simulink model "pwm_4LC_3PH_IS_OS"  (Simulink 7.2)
settings: Solver=ode3  SolverMode=SingleTasking  StartTime=0.0  StopTime=0.1  FixedStep=10e-6  MaxStep=1e-4  RelTol=1e-3

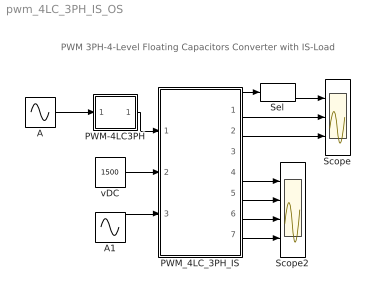
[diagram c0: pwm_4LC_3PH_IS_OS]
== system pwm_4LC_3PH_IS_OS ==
  note: PWM 3PH-4-Level Floating Capacitors Converter with IS-Load
  A : Sin  Amplitude=.9  Frequency=2*pi*50  Phase="[0  -2*pi/3  -4*pi/3]"  SampleTime=0
  A1 : Sin  Amplitude=500  Frequency=2*pi*50  Phase="[0  -2*pi/3 ]"  SampleTime=0
  PWM-4LC3PH : Subsystem  mask(PWM-4LC3PH){FT=900, PHT1=0, PHT2=-120, PHT3=-240, DT=1e-6}
      mask prompts: FT "Frequency of Trian Sig."; PHT1 "Phase Angle of 1st Trian. Sig."; PHT2 "Phase Angle of 2nd Trian. Sig."; PHT3 "Phase Angle of 3rd Trian. Sig."; DT "Dead Time"
  PWM_4LC_3PH_IS : Subsystem  mask(pwm_4LC_3PH_IS_OS){C1=10e-3, VC10=2*1500/3, C2=10e-3, VC20=1500/3}
      mask prompts: C1 "Cap C1"; VC10 "Initial Cap Voltage VC10"; C2 "Cap C2"; VC20 "Initial Cap Voltage VC20"
      mask help: Open Source 4-Level FC PWM 3PH Converter with IS load Input Vector u: u[0]= L4LC1_TD1.gate u[1]= L4LC1_TD2.gate u[2]= L4LC1_TD3.gate u[3]= L4LC1_TD4.gate u[4]= L4LC1_TD5.gate u[5]= L4LC1_TD6.gate u[6]= L4LC2_TD1.gate u[7]= L4LC2_TD2.gate u[8]= L4LC2_TD3.gate u[9]= L4LC2_TD4.gate u[10]= L4LC2_TD5.gate u[11]= L4LC2_TD6.gate u[12]= L4LC3_TD1.gate u[13]= L4LC3_TD2.gate u[14]= L4LC3_TD3.gate u[15]= L4LC3_TD4.gate u[15]= L4LC3_TD5.gate u[17]= L4LC3_TD6.gate u[18]= VDC u[19]= IA, Phase A Load Current as AC Current source u[20]= IB, Phase B Load Current as AC Current source Output Vector y: y[0]= Va.v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
  Scope : Scope  NumInputPorts=3
  Scope2 : Scope  NumInputPorts=4
  Sel : Selector  InputPortWidth=3  IndexOptions=Index vector (dialog)  Indices=[1 ]  OutputSizes=1
  vDC : Constant  Value=1500  OutDataType=sfix(16)  OutScaling=2^0
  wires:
  A/1 -> PWM-4LC3PH/1(In1)
  PWM-4LC3PH/1(Out1) -> PWM_4LC_3PH_IS/1(Sw)
  PWM_4LC_3PH_IS/1(vABC) -> Sel/1
  PWM_4LC_3PH_IS/2(iABC) -> Scope/2
  PWM_4LC_3PH_IS/3(vAB) -> Scope/3
  vDC/1 -> PWM_4LC_3PH_IS/2(vDC)
  A1/1 -> PWM_4LC_3PH_IS/3(i_AB)
  PWM_4LC_3PH_IS/4(iT1,iD1,vT1) -> Scope2/1
  PWM_4LC_3PH_IS/5(iT2,ID2,vT2) -> Scope2/2
  PWM_4LC_3PH_IS/6(iT3,iD3,vT3) -> Scope2/3
  PWM_4LC_3PH_IS/7(iDC1,IDC2) -> Scope2/4
  Sel/1 -> Scope/1

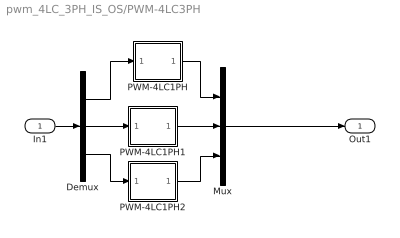
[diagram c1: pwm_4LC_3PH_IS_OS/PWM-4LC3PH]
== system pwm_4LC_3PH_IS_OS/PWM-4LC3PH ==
  In1 : Inport  OutDataType=sfix(16)  OutScaling=2^0
  Demux : Demux  Outputs=3
  Mux : Mux  Inputs=3
  PWM-4LC1PH : Subsystem  mask(PWM-4LC1PH){FT=FT, PHT1=PHT1, PHT2=PHT2, PHT3=PHT3, DT=DT}
      mask prompts: FT "Frequency of Trian Sig."; PHT1 "Phase Angle of 1st Trian. Sig."; PHT2 "Phase Angle of 2nd Trian. Sig."; PHT3 "Phase Angle of 3rd Trian. Sig."; DT "Dead Time"
      mask help: Pulse Width Modulation for 1 Phase 4 Level Floating Capacitor Converter
  PWM-4LC1PH1 : Subsystem  mask(PWM-4LC1PH){FT=FT, PHT1=PHT1, PHT2=PHT2, PHT3=PHT3, DT=DT}
      mask prompts: FT "Frequency of Trian Sig."; PHT1 "Phase Angle of 1st Trian. Sig."; PHT2 "Phase Angle of 2nd Trian. Sig."; PHT3 "Phase Angle of 3rd Trian. Sig."; DT "Dead Time"
      mask help: Pulse Width Modulation for 1 Phase 4 Level Floating Capacitor Converter
  PWM-4LC1PH2 : Subsystem  mask(PWM-4LC1PH){FT=FT, PHT1=PHT1, PHT2=PHT2, PHT3=PHT3, DT=DT}
      mask prompts: FT "Frequency of Trian Sig."; PHT1 "Phase Angle of 1st Trian. Sig."; PHT2 "Phase Angle of 2nd Trian. Sig."; PHT3 "Phase Angle of 3rd Trian. Sig."; DT "Dead Time"
      mask help: Pulse Width Modulation for 1 Phase 4 Level Floating Capacitor Converter
  Out1 : Outport
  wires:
  PWM-4LC1PH/1(Out1) -> Mux/1
  PWM-4LC1PH1/1(Out1) -> Mux/2
  PWM-4LC1PH2/1(Out1) -> Mux/3
  Demux/1 -> PWM-4LC1PH/1(In1)
  Demux/2 -> PWM-4LC1PH1/1(In1)
  Demux/3 -> PWM-4LC1PH2/1(In1)
  Mux/1 -> Out1/1
  In1/1 -> Demux/1

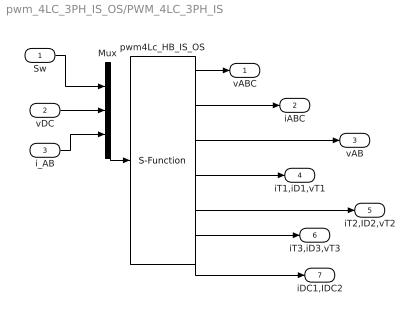
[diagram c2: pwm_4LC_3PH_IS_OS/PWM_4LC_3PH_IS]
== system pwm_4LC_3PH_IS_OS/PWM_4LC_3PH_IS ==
  Sw : Inport  OutDataType=sfix(16)  OutScaling=2^0
  vDC : Inport  Port=2  OutDataType=sfix(16)  OutScaling=2^0
  i_AB : Inport  Port=3  OutDataType=sfix(16)  OutScaling=2^0
  Mux : Mux  Inputs="[18  1  2]"
  pwm4Lc_HB_IS_OS : S-Function  FunctionName=s_pwm_4LC_3PH_IS_OS  Parameters="[C1  VC10  C2  VC20]"  EnableBusSupport=off
  vABC : Outport  OutDataType=sfix(16)  OutScaling=2^0
  iABC : Outport  Port=2  OutDataType=sfix(16)  OutScaling=2^0
  vAB : Outport  Port=3  OutDataType=sfix(16)  OutScaling=2^0
  iT1,iD1,vT1 : Outport  Port=4  OutDataType=sfix(16)  OutScaling=2^0
  iT2,ID2,vT2 : Outport  Port=5  OutDataType=sfix(16)  OutScaling=2^0
  iT3,iD3,vT3 : Outport  Port=6  OutDataType=sfix(16)  OutScaling=2^0
  iDC1,IDC2 : Outport  Port=7  OutDataType=sfix(16)  OutScaling=2^0
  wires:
  pwm4Lc_HB_IS_OS/7 -> iDC1,IDC2/1
  pwm4Lc_HB_IS_OS/2 -> iABC/1
  pwm4Lc_HB_IS_OS/1 -> vABC/1
  i_AB/1 -> Mux/3
  Mux/1 -> pwm4Lc_HB_IS_OS/1
  vDC/1 -> Mux/2
  Sw/1 -> Mux/1
  pwm4Lc_HB_IS_OS/3 -> vAB/1
  pwm4Lc_HB_IS_OS/4 -> iT1,iD1,vT1/1
  pwm4Lc_HB_IS_OS/5 -> iT2,ID2,vT2/1
  pwm4Lc_HB_IS_OS/6 -> iT3,iD3,vT3/1

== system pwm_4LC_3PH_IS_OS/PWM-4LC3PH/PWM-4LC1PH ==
  In1 : Inport  OutDataType=sfix(16)  OutScaling=2^0
  Mux : Mux  Inputs=6
  PWM-2L-1PH : Subsystem  mask(PWM-2L-1PH){FT=FT, PHT=PHT1, DT=DT}
      mask prompts: FT "Triangular Frequency"; PHT "Trian. Phase Angle (Degree)"; DT "Dead Time"
      mask help: Pulse Width Modulation for 1 Phase Converter
  PWM-2L-1PH1 : Subsystem  mask(PWM-2L-1PH){FT=FT, PHT=PHT2, DT=DT}
      mask prompts: FT "Triangular Frequency"; PHT "Trian. Phase Angle (Degree)"; DT "Dead Time"
      mask help: Pulse Width Modulation for 1 Phase Converter
  PWM-2L-1PH2 : Subsystem  mask(PWM-2L-1PH){FT=FT, PHT=PHT3, DT=DT}
      mask prompts: FT "Triangular Frequency"; PHT "Trian. Phase Angle (Degree)"; DT "Dead Time"
      mask help: Pulse Width Modulation for 1 Phase Converter
  Out1 : Outport
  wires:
  PWM-2L-1PH/1(Out1) -> Mux/1
  PWM-2L-1PH1/1(Out1) -> Mux/2
  PWM-2L-1PH1/2(Out2) -> Mux/5
  PWM-2L-1PH2/1(Out1) -> Mux/3
  PWM-2L-1PH2/2(Out2) -> Mux/4
  Mux/1 -> Out1/1
  In1/1 -> PWM-2L-1PH2/1(In1), PWM-2L-1PH1/1(In1), PWM-2L-1PH/1(In1)
  PWM-2L-1PH/2(Out2) -> Mux/6

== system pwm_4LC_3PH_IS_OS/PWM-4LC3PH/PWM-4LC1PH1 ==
  In1 : Inport  OutDataType=sfix(16)  OutScaling=2^0
  Mux : Mux  Inputs=6
  PWM-2L-1PH : Subsystem  mask(PWM-2L-1PH){FT=FT, PHT=PHT1, DT=DT}
      mask prompts: FT "Triangular Frequency"; PHT "Trian. Phase Angle (Degree)"; DT "Dead Time"
      mask help: Pulse Width Modulation for 1 Phase Converter
  PWM-2L-1PH1 : Subsystem  mask(PWM-2L-1PH){FT=FT, PHT=PHT2, DT=DT}
      mask prompts: FT "Triangular Frequency"; PHT "Trian. Phase Angle (Degree)"; DT "Dead Time"
      mask help: Pulse Width Modulation for 1 Phase Converter
  PWM-2L-1PH2 : Subsystem  mask(PWM-2L-1PH){FT=FT, PHT=PHT3, DT=DT}
      mask prompts: FT "Triangular Frequency"; PHT "Trian. Phase Angle (Degree)"; DT "Dead Time"
      mask help: Pulse Width Modulation for 1 Phase Converter
  Out1 : Outport
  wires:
  PWM-2L-1PH/2(Out2) -> Mux/6
  In1/1 -> PWM-2L-1PH/1(In1), PWM-2L-1PH1/1(In1), PWM-2L-1PH2/1(In1)
  Mux/1 -> Out1/1
  PWM-2L-1PH2/2(Out2) -> Mux/4
  PWM-2L-1PH2/1(Out1) -> Mux/3
  PWM-2L-1PH1/2(Out2) -> Mux/5
  PWM-2L-1PH1/1(Out1) -> Mux/2
  PWM-2L-1PH/1(Out1) -> Mux/1

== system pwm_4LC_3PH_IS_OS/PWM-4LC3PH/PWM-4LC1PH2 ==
  In1 : Inport  OutDataType=sfix(16)  OutScaling=2^0
  Mux : Mux  Inputs=6
  PWM-2L-1PH : Subsystem  mask(PWM-2L-1PH){FT=FT, PHT=PHT1, DT=DT}
      mask prompts: FT "Triangular Frequency"; PHT "Trian. Phase Angle (Degree)"; DT "Dead Time"
      mask help: Pulse Width Modulation for 1 Phase Converter
  PWM-2L-1PH1 : Subsystem  mask(PWM-2L-1PH){FT=FT, PHT=PHT2, DT=DT}
      mask prompts: FT "Triangular Frequency"; PHT "Trian. Phase Angle (Degree)"; DT "Dead Time"
      mask help: Pulse Width Modulation for 1 Phase Converter
  PWM-2L-1PH2 : Subsystem  mask(PWM-2L-1PH){FT=FT, PHT=PHT3, DT=DT}
      mask prompts: FT "Triangular Frequency"; PHT "Trian. Phase Angle (Degree)"; DT "Dead Time"
      mask help: Pulse Width Modulation for 1 Phase Converter
  Out1 : Outport
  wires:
  PWM-2L-1PH/1(Out1) -> Mux/1
  PWM-2L-1PH1/1(Out1) -> Mux/2
  PWM-2L-1PH1/2(Out2) -> Mux/5
  PWM-2L-1PH2/1(Out1) -> Mux/3
  PWM-2L-1PH2/2(Out2) -> Mux/4
  Mux/1 -> Out1/1
  In1/1 -> PWM-2L-1PH2/1(In1), PWM-2L-1PH1/1(In1), PWM-2L-1PH/1(In1)
  PWM-2L-1PH/2(Out2) -> Mux/6

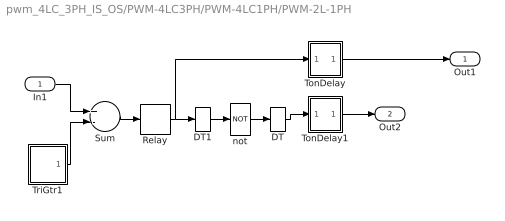
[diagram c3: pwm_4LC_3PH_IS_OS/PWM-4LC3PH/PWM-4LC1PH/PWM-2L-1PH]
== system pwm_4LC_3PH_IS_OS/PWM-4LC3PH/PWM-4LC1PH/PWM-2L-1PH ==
  In1 : Inport  OutDataType=sfix(16)  OutScaling=2^0
  DT : DataTypeConversion
  DT1 : DataTypeConversion
  Relay : Relay  OutDataType=sfix(16)  OutScaling=2^0
  Sum : Sum  Inputs=+-  OutDataType=sfix(16)  OutScaling=2^0
  TonDelay : Subsystem  mask(TonDelay){DT=DT}
      mask prompts: DT "Dead Time"
      mask help: Turn on dead time to protect against short circuit of the converter leg
  TonDelay1 : Subsystem  mask(TonDelay){DT=DT}
      mask prompts: DT "Dead Time"
      mask help: Turn on dead time to protect against short circuit of the converter leg
  TriGtr1 : Subsystem  mask(TriGtr){T=1/FT, Td=PHT/FT/360}
      mask prompts: T "Period Time"; Td "Time Delay"
      mask help: Triangular Wave Generator with variable time delay
  not : Logic  Operator=NOT  Inputs=1
  Out1 : Outport  InitialOutput=0
  Out2 : Outport  Port=2  InitialOutput=0
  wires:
  DT1/1 -> not/1
  DT/1 -> TonDelay1/1(s1)
  In1/1 -> Sum/1
  TriGtr1/1(O) -> Sum/2
  Sum/1 -> Relay/1
  not/1 -> DT/1
  TonDelay1/1(s1d) -> Out2/1
  Relay/1 -> DT1/1, TonDelay/1(s1)
  TonDelay/1(s1d) -> Out1/1

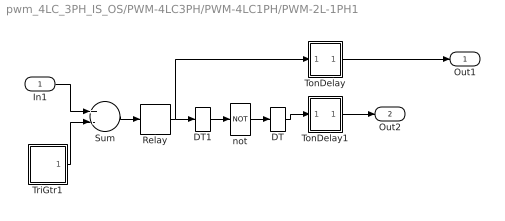
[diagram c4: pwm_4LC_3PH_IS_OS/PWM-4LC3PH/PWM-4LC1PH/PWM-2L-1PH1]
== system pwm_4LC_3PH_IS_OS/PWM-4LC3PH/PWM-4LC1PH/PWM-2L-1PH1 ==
  In1 : Inport  OutDataType=sfix(16)  OutScaling=2^0
  DT : DataTypeConversion
  DT1 : DataTypeConversion
  Relay : Relay  OutDataType=sfix(16)  OutScaling=2^0
  Sum : Sum  Inputs=+-  OutDataType=sfix(16)  OutScaling=2^0
  TonDelay : Subsystem  mask(TonDelay){DT=DT}
      mask prompts: DT "Dead Time"
      mask help: Turn on dead time to protect against short circuit of the converter leg
  TonDelay1 : Subsystem  mask(TonDelay){DT=DT}
      mask prompts: DT "Dead Time"
      mask help: Turn on dead time to protect against short circuit of the converter leg
  TriGtr1 : Subsystem  mask(TriGtr){T=1/FT, Td=PHT/FT/360}
      mask prompts: T "Period Time"; Td "Time Delay"
      mask help: Triangular Wave Generator with variable time delay
  not : Logic  Operator=NOT  Inputs=1
  Out1 : Outport  InitialOutput=0
  Out2 : Outport  Port=2  InitialOutput=0
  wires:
  TonDelay/1(s1d) -> Out1/1
  Relay/1 -> TonDelay/1(s1), DT1/1
  TonDelay1/1(s1d) -> Out2/1
  not/1 -> DT/1
  Sum/1 -> Relay/1
  TriGtr1/1(O) -> Sum/2
  In1/1 -> Sum/1
  DT/1 -> TonDelay1/1(s1)
  DT1/1 -> not/1

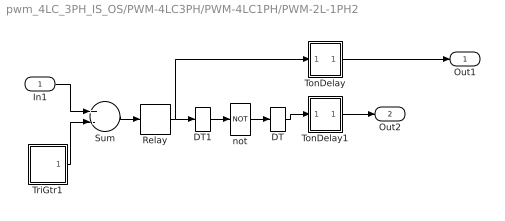
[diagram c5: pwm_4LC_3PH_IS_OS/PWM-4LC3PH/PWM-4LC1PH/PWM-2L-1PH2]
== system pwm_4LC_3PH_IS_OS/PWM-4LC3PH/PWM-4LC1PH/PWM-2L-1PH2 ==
  In1 : Inport  OutDataType=sfix(16)  OutScaling=2^0
  DT : DataTypeConversion
  DT1 : DataTypeConversion
  Relay : Relay  OutDataType=sfix(16)  OutScaling=2^0
  Sum : Sum  Inputs=+-  OutDataType=sfix(16)  OutScaling=2^0
  TonDelay : Subsystem  mask(TonDelay){DT=DT}
      mask prompts: DT "Dead Time"
      mask help: Turn on dead time to protect against short circuit of the converter leg
  TonDelay1 : Subsystem  mask(TonDelay){DT=DT}
      mask prompts: DT "Dead Time"
      mask help: Turn on dead time to protect against short circuit of the converter leg
  TriGtr1 : Subsystem  mask(TriGtr){T=1/FT, Td=PHT/FT/360}
      mask prompts: T "Period Time"; Td "Time Delay"
      mask help: Triangular Wave Generator with variable time delay
  not : Logic  Operator=NOT  Inputs=1
  Out1 : Outport  InitialOutput=0
  Out2 : Outport  Port=2  InitialOutput=0
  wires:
  DT1/1 -> not/1
  DT/1 -> TonDelay1/1(s1)
  In1/1 -> Sum/1
  TriGtr1/1(O) -> Sum/2
  Sum/1 -> Relay/1
  not/1 -> DT/1
  TonDelay1/1(s1d) -> Out2/1
  Relay/1 -> DT1/1, TonDelay/1(s1)
  TonDelay/1(s1d) -> Out1/1

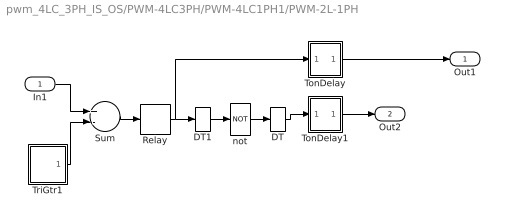
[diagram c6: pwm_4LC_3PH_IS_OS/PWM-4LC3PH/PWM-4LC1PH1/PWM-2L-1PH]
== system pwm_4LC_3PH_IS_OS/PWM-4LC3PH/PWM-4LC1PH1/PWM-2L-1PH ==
  In1 : Inport  OutDataType=sfix(16)  OutScaling=2^0
  DT : DataTypeConversion
  DT1 : DataTypeConversion
  Relay : Relay  OutDataType=sfix(16)  OutScaling=2^0
  Sum : Sum  Inputs=+-  OutDataType=sfix(16)  OutScaling=2^0
  TonDelay : Subsystem  mask(TonDelay){DT=DT}
      mask prompts: DT "Dead Time"
      mask help: Turn on dead time to protect against short circuit of the converter leg
  TonDelay1 : Subsystem  mask(TonDelay){DT=DT}
      mask prompts: DT "Dead Time"
      mask help: Turn on dead time to protect against short circuit of the converter leg
  TriGtr1 : Subsystem  mask(TriGtr){T=1/FT, Td=PHT/FT/360}
      mask prompts: T "Period Time"; Td "Time Delay"
      mask help: Triangular Wave Generator with variable time delay
  not : Logic  Operator=NOT  Inputs=1
  Out1 : Outport  InitialOutput=0
  Out2 : Outport  Port=2  InitialOutput=0
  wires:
  TonDelay/1(s1d) -> Out1/1
  Relay/1 -> TonDelay/1(s1), DT1/1
  TonDelay1/1(s1d) -> Out2/1
  not/1 -> DT/1
  Sum/1 -> Relay/1
  TriGtr1/1(O) -> Sum/2
  In1/1 -> Sum/1
  DT/1 -> TonDelay1/1(s1)
  DT1/1 -> not/1

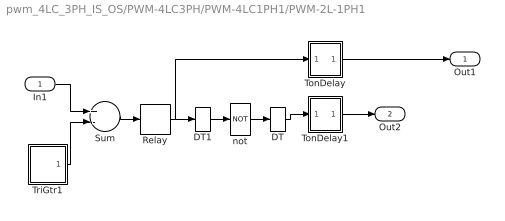
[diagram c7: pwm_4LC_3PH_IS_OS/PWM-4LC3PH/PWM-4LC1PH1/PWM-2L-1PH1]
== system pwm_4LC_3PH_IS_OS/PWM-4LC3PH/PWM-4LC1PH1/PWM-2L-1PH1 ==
  In1 : Inport  OutDataType=sfix(16)  OutScaling=2^0
  DT : DataTypeConversion
  DT1 : DataTypeConversion
  Relay : Relay  OutDataType=sfix(16)  OutScaling=2^0
  Sum : Sum  Inputs=+-  OutDataType=sfix(16)  OutScaling=2^0
  TonDelay : Subsystem  mask(TonDelay){DT=DT}
      mask prompts: DT "Dead Time"
      mask help: Turn on dead time to protect against short circuit of the converter leg
  TonDelay1 : Subsystem  mask(TonDelay){DT=DT}
      mask prompts: DT "Dead Time"
      mask help: Turn on dead time to protect against short circuit of the converter leg
  TriGtr1 : Subsystem  mask(TriGtr){T=1/FT, Td=PHT/FT/360}
      mask prompts: T "Period Time"; Td "Time Delay"
      mask help: Triangular Wave Generator with variable time delay
  not : Logic  Operator=NOT  Inputs=1
  Out1 : Outport  InitialOutput=0
  Out2 : Outport  Port=2  InitialOutput=0
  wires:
  DT1/1 -> not/1
  DT/1 -> TonDelay1/1(s1)
  In1/1 -> Sum/1
  TriGtr1/1(O) -> Sum/2
  Sum/1 -> Relay/1
  not/1 -> DT/1
  TonDelay1/1(s1d) -> Out2/1
  Relay/1 -> DT1/1, TonDelay/1(s1)
  TonDelay/1(s1d) -> Out1/1

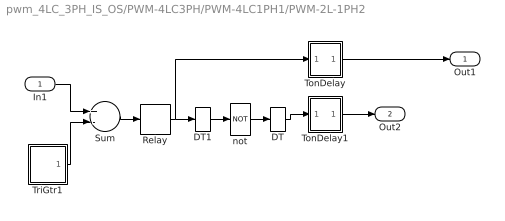
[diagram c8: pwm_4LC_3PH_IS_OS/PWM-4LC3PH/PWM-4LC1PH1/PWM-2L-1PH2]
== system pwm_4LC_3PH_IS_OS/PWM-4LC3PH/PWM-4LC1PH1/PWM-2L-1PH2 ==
  In1 : Inport  OutDataType=sfix(16)  OutScaling=2^0
  DT : DataTypeConversion
  DT1 : DataTypeConversion
  Relay : Relay  OutDataType=sfix(16)  OutScaling=2^0
  Sum : Sum  Inputs=+-  OutDataType=sfix(16)  OutScaling=2^0
  TonDelay : Subsystem  mask(TonDelay){DT=DT}
      mask prompts: DT "Dead Time"
      mask help: Turn on dead time to protect against short circuit of the converter leg
  TonDelay1 : Subsystem  mask(TonDelay){DT=DT}
      mask prompts: DT "Dead Time"
      mask help: Turn on dead time to protect against short circuit of the converter leg
  TriGtr1 : Subsystem  mask(TriGtr){T=1/FT, Td=PHT/FT/360}
      mask prompts: T "Period Time"; Td "Time Delay"
      mask help: Triangular Wave Generator with variable time delay
  not : Logic  Operator=NOT  Inputs=1
  Out1 : Outport  InitialOutput=0
  Out2 : Outport  Port=2  InitialOutput=0
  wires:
  TonDelay/1(s1d) -> Out1/1
  Relay/1 -> TonDelay/1(s1), DT1/1
  TonDelay1/1(s1d) -> Out2/1
  not/1 -> DT/1
  Sum/1 -> Relay/1
  TriGtr1/1(O) -> Sum/2
  In1/1 -> Sum/1
  DT/1 -> TonDelay1/1(s1)
  DT1/1 -> not/1

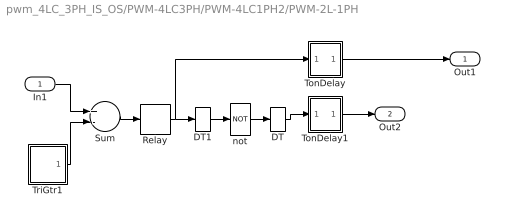
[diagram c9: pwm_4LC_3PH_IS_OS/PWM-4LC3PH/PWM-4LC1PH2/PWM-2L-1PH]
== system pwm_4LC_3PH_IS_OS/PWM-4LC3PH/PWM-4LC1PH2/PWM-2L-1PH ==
  In1 : Inport  OutDataType=sfix(16)  OutScaling=2^0
  DT : DataTypeConversion
  DT1 : DataTypeConversion
  Relay : Relay  OutDataType=sfix(16)  OutScaling=2^0
  Sum : Sum  Inputs=+-  OutDataType=sfix(16)  OutScaling=2^0
  TonDelay : Subsystem  mask(TonDelay){DT=DT}
      mask prompts: DT "Dead Time"
      mask help: Turn on dead time to protect against short circuit of the converter leg
  TonDelay1 : Subsystem  mask(TonDelay){DT=DT}
      mask prompts: DT "Dead Time"
      mask help: Turn on dead time to protect against short circuit of the converter leg
  TriGtr1 : Subsystem  mask(TriGtr){T=1/FT, Td=PHT/FT/360}
      mask prompts: T "Period Time"; Td "Time Delay"
      mask help: Triangular Wave Generator with variable time delay
  not : Logic  Operator=NOT  Inputs=1
  Out1 : Outport  InitialOutput=0
  Out2 : Outport  Port=2  InitialOutput=0
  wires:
  DT1/1 -> not/1
  DT/1 -> TonDelay1/1(s1)
  In1/1 -> Sum/1
  TriGtr1/1(O) -> Sum/2
  Sum/1 -> Relay/1
  not/1 -> DT/1
  TonDelay1/1(s1d) -> Out2/1
  Relay/1 -> DT1/1, TonDelay/1(s1)
  TonDelay/1(s1d) -> Out1/1

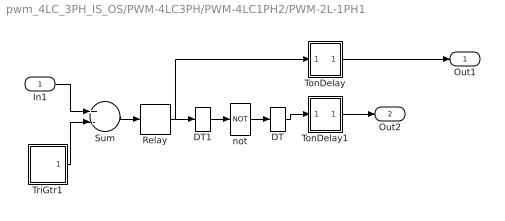
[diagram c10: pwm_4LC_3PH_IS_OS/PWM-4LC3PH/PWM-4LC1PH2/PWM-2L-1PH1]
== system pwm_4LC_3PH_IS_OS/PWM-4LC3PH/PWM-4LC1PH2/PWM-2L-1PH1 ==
  In1 : Inport  OutDataType=sfix(16)  OutScaling=2^0
  DT : DataTypeConversion
  DT1 : DataTypeConversion
  Relay : Relay  OutDataType=sfix(16)  OutScaling=2^0
  Sum : Sum  Inputs=+-  OutDataType=sfix(16)  OutScaling=2^0
  TonDelay : Subsystem  mask(TonDelay){DT=DT}
      mask prompts: DT "Dead Time"
      mask help: Turn on dead time to protect against short circuit of the converter leg
  TonDelay1 : Subsystem  mask(TonDelay){DT=DT}
      mask prompts: DT "Dead Time"
      mask help: Turn on dead time to protect against short circuit of the converter leg
  TriGtr1 : Subsystem  mask(TriGtr){T=1/FT, Td=PHT/FT/360}
      mask prompts: T "Period Time"; Td "Time Delay"
      mask help: Triangular Wave Generator with variable time delay
  not : Logic  Operator=NOT  Inputs=1
  Out1 : Outport  InitialOutput=0
  Out2 : Outport  Port=2  InitialOutput=0
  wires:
  TonDelay/1(s1d) -> Out1/1
  Relay/1 -> TonDelay/1(s1), DT1/1
  TonDelay1/1(s1d) -> Out2/1
  not/1 -> DT/1
  Sum/1 -> Relay/1
  TriGtr1/1(O) -> Sum/2
  In1/1 -> Sum/1
  DT/1 -> TonDelay1/1(s1)
  DT1/1 -> not/1

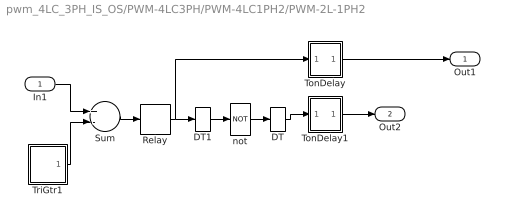
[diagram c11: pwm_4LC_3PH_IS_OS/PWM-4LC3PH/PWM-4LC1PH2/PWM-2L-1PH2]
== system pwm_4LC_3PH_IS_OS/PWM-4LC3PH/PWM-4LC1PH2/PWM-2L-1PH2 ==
  In1 : Inport  OutDataType=sfix(16)  OutScaling=2^0
  DT : DataTypeConversion
  DT1 : DataTypeConversion
  Relay : Relay  OutDataType=sfix(16)  OutScaling=2^0
  Sum : Sum  Inputs=+-  OutDataType=sfix(16)  OutScaling=2^0
  TonDelay : Subsystem  mask(TonDelay){DT=DT}
      mask prompts: DT "Dead Time"
      mask help: Turn on dead time to protect against short circuit of the converter leg
  TonDelay1 : Subsystem  mask(TonDelay){DT=DT}
      mask prompts: DT "Dead Time"
      mask help: Turn on dead time to protect against short circuit of the converter leg
  TriGtr1 : Subsystem  mask(TriGtr){T=1/FT, Td=PHT/FT/360}
      mask prompts: T "Period Time"; Td "Time Delay"
      mask help: Triangular Wave Generator with variable time delay
  not : Logic  Operator=NOT  Inputs=1
  Out1 : Outport  InitialOutput=0
  Out2 : Outport  Port=2  InitialOutput=0
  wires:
  DT1/1 -> not/1
  DT/1 -> TonDelay1/1(s1)
  In1/1 -> Sum/1
  TriGtr1/1(O) -> Sum/2
  Sum/1 -> Relay/1
  not/1 -> DT/1
  TonDelay1/1(s1d) -> Out2/1
  Relay/1 -> DT1/1, TonDelay/1(s1)
  TonDelay/1(s1d) -> Out1/1

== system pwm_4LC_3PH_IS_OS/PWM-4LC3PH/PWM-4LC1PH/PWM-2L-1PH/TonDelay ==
  s1 : Inport  Orientation=down  OutDataType=sfix(16)  OutScaling=2^0
  Int : Integrator  ExternalReset=falling
  Rel1 : Relay  OnSwitchValue=DT  OutDataType=sfix(16)  OutScaling=2^0
  s1d : Outport  InitialOutput=0
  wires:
  Int/1 -> Rel1/1
  s1/1 -> Int/2, Int/1
  Rel1/1 -> s1d/1

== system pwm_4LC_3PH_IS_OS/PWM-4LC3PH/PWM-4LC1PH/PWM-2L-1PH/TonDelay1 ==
  s1 : Inport  Orientation=down  OutDataType=sfix(16)  OutScaling=2^0
  Int : Integrator  ExternalReset=falling
  Rel1 : Relay  OnSwitchValue=DT  OutDataType=sfix(16)  OutScaling=2^0
  s1d : Outport  InitialOutput=0
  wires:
  Int/1 -> Rel1/1
  s1/1 -> Int/2, Int/1
  Rel1/1 -> s1d/1

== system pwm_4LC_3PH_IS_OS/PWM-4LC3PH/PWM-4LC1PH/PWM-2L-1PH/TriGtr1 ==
  Clock : Clock
  S1 : Subsystem
  Sum : Sum  OutDataType=sfix(16)  OutScaling=2^0
  T : Constant  Value=T  OutDataType=sfix(16)  OutScaling=2^0
  Td : Constant  Value=Td  OutDataType=sfix(16)  OutScaling=2^0
  mod : Math  Operator=mod
  O : Outport  InitialOutput=0
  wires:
  mod/1 -> S1/1(I1)
  S1/1(O1) -> O/1
  Clock/1 -> Sum/1
  T/1 -> mod/2
  Sum/1 -> mod/1
  Td/1 -> Sum/2

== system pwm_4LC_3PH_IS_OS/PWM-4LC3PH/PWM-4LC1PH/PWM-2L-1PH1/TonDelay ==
  s1 : Inport  Orientation=down  OutDataType=sfix(16)  OutScaling=2^0
  Int : Integrator  ExternalReset=falling
  Rel1 : Relay  OnSwitchValue=DT  OutDataType=sfix(16)  OutScaling=2^0
  s1d : Outport  InitialOutput=0
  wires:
  Rel1/1 -> s1d/1
  s1/1 -> Int/1, Int/2
  Int/1 -> Rel1/1

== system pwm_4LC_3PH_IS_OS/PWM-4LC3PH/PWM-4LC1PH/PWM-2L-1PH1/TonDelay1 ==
  s1 : Inport  Orientation=down  OutDataType=sfix(16)  OutScaling=2^0
  Int : Integrator  ExternalReset=falling
  Rel1 : Relay  OnSwitchValue=DT  OutDataType=sfix(16)  OutScaling=2^0
  s1d : Outport  InitialOutput=0
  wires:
  Rel1/1 -> s1d/1
  s1/1 -> Int/1, Int/2
  Int/1 -> Rel1/1

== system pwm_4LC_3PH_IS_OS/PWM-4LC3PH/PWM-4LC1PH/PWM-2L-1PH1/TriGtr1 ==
  Clock : Clock
  S1 : Subsystem
  Sum : Sum  OutDataType=sfix(16)  OutScaling=2^0
  T : Constant  Value=T  OutDataType=sfix(16)  OutScaling=2^0
  Td : Constant  Value=Td  OutDataType=sfix(16)  OutScaling=2^0
  mod : Math  Operator=mod
  O : Outport  InitialOutput=0
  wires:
  Td/1 -> Sum/2
  Sum/1 -> mod/1
  T/1 -> mod/2
  Clock/1 -> Sum/1
  S1/1(O1) -> O/1
  mod/1 -> S1/1(I1)

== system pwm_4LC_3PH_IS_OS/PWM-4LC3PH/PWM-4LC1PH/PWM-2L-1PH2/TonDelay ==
  s1 : Inport  Orientation=down  OutDataType=sfix(16)  OutScaling=2^0
  Int : Integrator  ExternalReset=falling
  Rel1 : Relay  OnSwitchValue=DT  OutDataType=sfix(16)  OutScaling=2^0
  s1d : Outport  InitialOutput=0
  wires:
  Int/1 -> Rel1/1
  s1/1 -> Int/2, Int/1
  Rel1/1 -> s1d/1

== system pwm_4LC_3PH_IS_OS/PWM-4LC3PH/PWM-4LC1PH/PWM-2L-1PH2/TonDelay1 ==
  s1 : Inport  Orientation=down  OutDataType=sfix(16)  OutScaling=2^0
  Int : Integrator  ExternalReset=falling
  Rel1 : Relay  OnSwitchValue=DT  OutDataType=sfix(16)  OutScaling=2^0
  s1d : Outport  InitialOutput=0
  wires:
  Int/1 -> Rel1/1
  s1/1 -> Int/2, Int/1
  Rel1/1 -> s1d/1

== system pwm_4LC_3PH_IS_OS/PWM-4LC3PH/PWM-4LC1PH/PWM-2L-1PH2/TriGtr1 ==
  Clock : Clock
  S1 : Subsystem
  Sum : Sum  OutDataType=sfix(16)  OutScaling=2^0
  T : Constant  Value=T  OutDataType=sfix(16)  OutScaling=2^0
  Td : Constant  Value=Td  OutDataType=sfix(16)  OutScaling=2^0
  mod : Math  Operator=mod
  O : Outport  InitialOutput=0
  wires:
  mod/1 -> S1/1(I1)
  S1/1(O1) -> O/1
  Clock/1 -> Sum/1
  T/1 -> mod/2
  Sum/1 -> mod/1
  Td/1 -> Sum/2

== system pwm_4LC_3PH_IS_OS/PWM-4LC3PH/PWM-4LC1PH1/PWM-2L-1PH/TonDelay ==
  s1 : Inport  Orientation=down  OutDataType=sfix(16)  OutScaling=2^0
  Int : Integrator  ExternalReset=falling
  Rel1 : Relay  OnSwitchValue=DT  OutDataType=sfix(16)  OutScaling=2^0
  s1d : Outport  InitialOutput=0
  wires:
  Rel1/1 -> s1d/1
  s1/1 -> Int/1, Int/2
  Int/1 -> Rel1/1

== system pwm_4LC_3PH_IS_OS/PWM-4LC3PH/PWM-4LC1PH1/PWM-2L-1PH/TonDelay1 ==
  s1 : Inport  Orientation=down  OutDataType=sfix(16)  OutScaling=2^0
  Int : Integrator  ExternalReset=falling
  Rel1 : Relay  OnSwitchValue=DT  OutDataType=sfix(16)  OutScaling=2^0
  s1d : Outport  InitialOutput=0
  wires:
  Rel1/1 -> s1d/1
  s1/1 -> Int/1, Int/2
  Int/1 -> Rel1/1

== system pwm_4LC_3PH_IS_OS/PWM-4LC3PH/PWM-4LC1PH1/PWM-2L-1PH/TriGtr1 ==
  Clock : Clock
  S1 : Subsystem
  Sum : Sum  OutDataType=sfix(16)  OutScaling=2^0
  T : Constant  Value=T  OutDataType=sfix(16)  OutScaling=2^0
  Td : Constant  Value=Td  OutDataType=sfix(16)  OutScaling=2^0
  mod : Math  Operator=mod
  O : Outport  InitialOutput=0
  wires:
  Td/1 -> Sum/2
  Sum/1 -> mod/1
  T/1 -> mod/2
  Clock/1 -> Sum/1
  S1/1(O1) -> O/1
  mod/1 -> S1/1(I1)

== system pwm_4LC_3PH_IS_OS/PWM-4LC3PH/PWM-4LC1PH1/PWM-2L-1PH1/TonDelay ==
  s1 : Inport  Orientation=down  OutDataType=sfix(16)  OutScaling=2^0
  Int : Integrator  ExternalReset=falling
  Rel1 : Relay  OnSwitchValue=DT  OutDataType=sfix(16)  OutScaling=2^0
  s1d : Outport  InitialOutput=0
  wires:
  Int/1 -> Rel1/1
  s1/1 -> Int/2, Int/1
  Rel1/1 -> s1d/1

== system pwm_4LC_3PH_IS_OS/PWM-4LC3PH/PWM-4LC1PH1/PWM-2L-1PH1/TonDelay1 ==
  s1 : Inport  Orientation=down  OutDataType=sfix(16)  OutScaling=2^0
  Int : Integrator  ExternalReset=falling
  Rel1 : Relay  OnSwitchValue=DT  OutDataType=sfix(16)  OutScaling=2^0
  s1d : Outport  InitialOutput=0
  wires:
  Int/1 -> Rel1/1
  s1/1 -> Int/2, Int/1
  Rel1/1 -> s1d/1

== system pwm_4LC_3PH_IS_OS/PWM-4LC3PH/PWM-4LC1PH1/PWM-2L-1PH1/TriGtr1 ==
  Clock : Clock
  S1 : Subsystem
  Sum : Sum  OutDataType=sfix(16)  OutScaling=2^0
  T : Constant  Value=T  OutDataType=sfix(16)  OutScaling=2^0
  Td : Constant  Value=Td  OutDataType=sfix(16)  OutScaling=2^0
  mod : Math  Operator=mod
  O : Outport  InitialOutput=0
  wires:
  mod/1 -> S1/1(I1)
  S1/1(O1) -> O/1
  Clock/1 -> Sum/1
  T/1 -> mod/2
  Sum/1 -> mod/1
  Td/1 -> Sum/2

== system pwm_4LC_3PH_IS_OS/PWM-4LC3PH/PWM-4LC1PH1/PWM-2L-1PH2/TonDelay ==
  s1 : Inport  Orientation=down  OutDataType=sfix(16)  OutScaling=2^0
  Int : Integrator  ExternalReset=falling
  Rel1 : Relay  OnSwitchValue=DT  OutDataType=sfix(16)  OutScaling=2^0
  s1d : Outport  InitialOutput=0
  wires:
  Rel1/1 -> s1d/1
  s1/1 -> Int/1, Int/2
  Int/1 -> Rel1/1

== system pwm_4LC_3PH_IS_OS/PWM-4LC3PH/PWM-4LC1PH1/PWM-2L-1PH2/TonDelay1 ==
  s1 : Inport  Orientation=down  OutDataType=sfix(16)  OutScaling=2^0
  Int : Integrator  ExternalReset=falling
  Rel1 : Relay  OnSwitchValue=DT  OutDataType=sfix(16)  OutScaling=2^0
  s1d : Outport  InitialOutput=0
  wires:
  Rel1/1 -> s1d/1
  s1/1 -> Int/1, Int/2
  Int/1 -> Rel1/1

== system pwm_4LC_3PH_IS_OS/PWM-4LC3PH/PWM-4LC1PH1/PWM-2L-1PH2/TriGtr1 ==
  Clock : Clock
  S1 : Subsystem
  Sum : Sum  OutDataType=sfix(16)  OutScaling=2^0
  T : Constant  Value=T  OutDataType=sfix(16)  OutScaling=2^0
  Td : Constant  Value=Td  OutDataType=sfix(16)  OutScaling=2^0
  mod : Math  Operator=mod
  O : Outport  InitialOutput=0
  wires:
  Td/1 -> Sum/2
  Sum/1 -> mod/1
  T/1 -> mod/2
  Clock/1 -> Sum/1
  S1/1(O1) -> O/1
  mod/1 -> S1/1(I1)

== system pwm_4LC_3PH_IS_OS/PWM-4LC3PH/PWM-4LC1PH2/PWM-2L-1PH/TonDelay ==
  s1 : Inport  Orientation=down  OutDataType=sfix(16)  OutScaling=2^0
  Int : Integrator  ExternalReset=falling
  Rel1 : Relay  OnSwitchValue=DT  OutDataType=sfix(16)  OutScaling=2^0
  s1d : Outport  InitialOutput=0
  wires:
  Int/1 -> Rel1/1
  s1/1 -> Int/2, Int/1
  Rel1/1 -> s1d/1

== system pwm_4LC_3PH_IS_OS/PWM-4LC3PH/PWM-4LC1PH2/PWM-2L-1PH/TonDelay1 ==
  s1 : Inport  Orientation=down  OutDataType=sfix(16)  OutScaling=2^0
  Int : Integrator  ExternalReset=falling
  Rel1 : Relay  OnSwitchValue=DT  OutDataType=sfix(16)  OutScaling=2^0
  s1d : Outport  InitialOutput=0
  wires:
  Int/1 -> Rel1/1
  s1/1 -> Int/2, Int/1
  Rel1/1 -> s1d/1

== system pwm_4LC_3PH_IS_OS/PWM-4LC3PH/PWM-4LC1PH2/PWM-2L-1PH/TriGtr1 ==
  Clock : Clock
  S1 : Subsystem
  Sum : Sum  OutDataType=sfix(16)  OutScaling=2^0
  T : Constant  Value=T  OutDataType=sfix(16)  OutScaling=2^0
  Td : Constant  Value=Td  OutDataType=sfix(16)  OutScaling=2^0
  mod : Math  Operator=mod
  O : Outport  InitialOutput=0
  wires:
  mod/1 -> S1/1(I1)
  S1/1(O1) -> O/1
  Clock/1 -> Sum/1
  T/1 -> mod/2
  Sum/1 -> mod/1
  Td/1 -> Sum/2

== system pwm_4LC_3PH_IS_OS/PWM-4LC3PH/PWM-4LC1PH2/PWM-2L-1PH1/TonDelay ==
  s1 : Inport  Orientation=down  OutDataType=sfix(16)  OutScaling=2^0
  Int : Integrator  ExternalReset=falling
  Rel1 : Relay  OnSwitchValue=DT  OutDataType=sfix(16)  OutScaling=2^0
  s1d : Outport  InitialOutput=0
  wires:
  Rel1/1 -> s1d/1
  s1/1 -> Int/1, Int/2
  Int/1 -> Rel1/1

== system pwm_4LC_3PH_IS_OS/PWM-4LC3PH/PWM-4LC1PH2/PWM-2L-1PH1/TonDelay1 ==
  s1 : Inport  Orientation=down  OutDataType=sfix(16)  OutScaling=2^0
  Int : Integrator  ExternalReset=falling
  Rel1 : Relay  OnSwitchValue=DT  OutDataType=sfix(16)  OutScaling=2^0
  s1d : Outport  InitialOutput=0
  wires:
  Rel1/1 -> s1d/1
  s1/1 -> Int/1, Int/2
  Int/1 -> Rel1/1

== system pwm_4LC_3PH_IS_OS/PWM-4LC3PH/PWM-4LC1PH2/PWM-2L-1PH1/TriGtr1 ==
  Clock : Clock
  S1 : Subsystem
  Sum : Sum  OutDataType=sfix(16)  OutScaling=2^0
  T : Constant  Value=T  OutDataType=sfix(16)  OutScaling=2^0
  Td : Constant  Value=Td  OutDataType=sfix(16)  OutScaling=2^0
  mod : Math  Operator=mod
  O : Outport  InitialOutput=0
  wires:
  Td/1 -> Sum/2
  Sum/1 -> mod/1
  T/1 -> mod/2
  Clock/1 -> Sum/1
  S1/1(O1) -> O/1
  mod/1 -> S1/1(I1)

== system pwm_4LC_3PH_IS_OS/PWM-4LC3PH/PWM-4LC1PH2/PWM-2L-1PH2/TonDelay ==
  s1 : Inport  Orientation=down  OutDataType=sfix(16)  OutScaling=2^0
  Int : Integrator  ExternalReset=falling
  Rel1 : Relay  OnSwitchValue=DT  OutDataType=sfix(16)  OutScaling=2^0
  s1d : Outport  InitialOutput=0
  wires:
  Int/1 -> Rel1/1
  s1/1 -> Int/2, Int/1
  Rel1/1 -> s1d/1

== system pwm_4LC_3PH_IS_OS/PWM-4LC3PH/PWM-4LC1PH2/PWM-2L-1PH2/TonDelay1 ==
  s1 : Inport  Orientation=down  OutDataType=sfix(16)  OutScaling=2^0
  Int : Integrator  ExternalReset=falling
  Rel1 : Relay  OnSwitchValue=DT  OutDataType=sfix(16)  OutScaling=2^0
  s1d : Outport  InitialOutput=0
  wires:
  Int/1 -> Rel1/1
  s1/1 -> Int/2, Int/1
  Rel1/1 -> s1d/1

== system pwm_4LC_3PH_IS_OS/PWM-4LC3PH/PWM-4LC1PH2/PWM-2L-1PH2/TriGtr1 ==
  Clock : Clock
  S1 : Subsystem
  Sum : Sum  OutDataType=sfix(16)  OutScaling=2^0
  T : Constant  Value=T  OutDataType=sfix(16)  OutScaling=2^0
  Td : Constant  Value=Td  OutDataType=sfix(16)  OutScaling=2^0
  mod : Math  Operator=mod
  O : Outport  InitialOutput=0
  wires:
  mod/1 -> S1/1(I1)
  S1/1(O1) -> O/1
  Clock/1 -> Sum/1
  T/1 -> mod/2
  Sum/1 -> mod/1
  Td/1 -> Sum/2

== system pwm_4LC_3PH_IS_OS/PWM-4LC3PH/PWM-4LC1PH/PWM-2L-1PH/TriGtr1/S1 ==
  I1 : Inport  OutDataType=sfix(16)  OutScaling=2^0
  Fcn : Fcn  Expr=u* (u <=T/4) * 4/T
  Fcn1 : Fcn  Expr="(  (u > T/4) && ( u <=3*T/4) )* ( 1 - (u-T/4) *4/T )"
  Fcn2 : Fcn  Expr=( (u > 3*T/4)&& (u<=T)) * ( ((u -3*T/4)* 4/T )-1 )
  Sum1 : Sum  Inputs=+++  OutDataType=sfix(16)  OutScaling=2^0
  O1 : Outport
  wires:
  Fcn2/1 -> Sum1/3
  Fcn1/1 -> Sum1/2
  Fcn/1 -> Sum1/1
  Sum1/1 -> O1/1
  I1/1 -> Fcn/1, Fcn2/1, Fcn1/1

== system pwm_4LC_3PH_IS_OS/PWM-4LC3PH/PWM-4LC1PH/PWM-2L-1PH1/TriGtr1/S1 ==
  I1 : Inport  OutDataType=sfix(16)  OutScaling=2^0
  Fcn : Fcn  Expr=u* (u <=T/4) * 4/T
  Fcn1 : Fcn  Expr="(  (u > T/4) && ( u <=3*T/4) )* ( 1 - (u-T/4) *4/T )"
  Fcn2 : Fcn  Expr=( (u > 3*T/4)&& (u<=T)) * ( ((u -3*T/4)* 4/T )-1 )
  Sum1 : Sum  Inputs=+++  OutDataType=sfix(16)  OutScaling=2^0
  O1 : Outport
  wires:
  I1/1 -> Fcn1/1, Fcn2/1, Fcn/1
  Sum1/1 -> O1/1
  Fcn/1 -> Sum1/1
  Fcn1/1 -> Sum1/2
  Fcn2/1 -> Sum1/3

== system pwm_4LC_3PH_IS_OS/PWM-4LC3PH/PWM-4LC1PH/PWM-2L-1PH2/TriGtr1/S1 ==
  I1 : Inport  OutDataType=sfix(16)  OutScaling=2^0
  Fcn : Fcn  Expr=u* (u <=T/4) * 4/T
  Fcn1 : Fcn  Expr="(  (u > T/4) && ( u <=3*T/4) )* ( 1 - (u-T/4) *4/T )"
  Fcn2 : Fcn  Expr=( (u > 3*T/4)&& (u<=T)) * ( ((u -3*T/4)* 4/T )-1 )
  Sum1 : Sum  Inputs=+++  OutDataType=sfix(16)  OutScaling=2^0
  O1 : Outport
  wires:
  Fcn2/1 -> Sum1/3
  Fcn1/1 -> Sum1/2
  Fcn/1 -> Sum1/1
  Sum1/1 -> O1/1
  I1/1 -> Fcn/1, Fcn2/1, Fcn1/1

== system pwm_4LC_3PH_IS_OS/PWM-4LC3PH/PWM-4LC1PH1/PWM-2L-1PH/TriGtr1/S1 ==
  I1 : Inport  OutDataType=sfix(16)  OutScaling=2^0
  Fcn : Fcn  Expr=u* (u <=T/4) * 4/T
  Fcn1 : Fcn  Expr="(  (u > T/4) && ( u <=3*T/4) )* ( 1 - (u-T/4) *4/T )"
  Fcn2 : Fcn  Expr=( (u > 3*T/4)&& (u<=T)) * ( ((u -3*T/4)* 4/T )-1 )
  Sum1 : Sum  Inputs=+++  OutDataType=sfix(16)  OutScaling=2^0
  O1 : Outport
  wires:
  I1/1 -> Fcn1/1, Fcn2/1, Fcn/1
  Sum1/1 -> O1/1
  Fcn/1 -> Sum1/1
  Fcn1/1 -> Sum1/2
  Fcn2/1 -> Sum1/3

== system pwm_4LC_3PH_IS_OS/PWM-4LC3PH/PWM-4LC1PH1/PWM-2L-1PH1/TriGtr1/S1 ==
  I1 : Inport  OutDataType=sfix(16)  OutScaling=2^0
  Fcn : Fcn  Expr=u* (u <=T/4) * 4/T
  Fcn1 : Fcn  Expr="(  (u > T/4) && ( u <=3*T/4) )* ( 1 - (u-T/4) *4/T )"
  Fcn2 : Fcn  Expr=( (u > 3*T/4)&& (u<=T)) * ( ((u -3*T/4)* 4/T )-1 )
  Sum1 : Sum  Inputs=+++  OutDataType=sfix(16)  OutScaling=2^0
  O1 : Outport
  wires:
  Fcn2/1 -> Sum1/3
  Fcn1/1 -> Sum1/2
  Fcn/1 -> Sum1/1
  Sum1/1 -> O1/1
  I1/1 -> Fcn/1, Fcn2/1, Fcn1/1

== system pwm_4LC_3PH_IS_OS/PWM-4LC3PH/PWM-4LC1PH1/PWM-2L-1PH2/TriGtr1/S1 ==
  I1 : Inport  OutDataType=sfix(16)  OutScaling=2^0
  Fcn : Fcn  Expr=u* (u <=T/4) * 4/T
  Fcn1 : Fcn  Expr="(  (u > T/4) && ( u <=3*T/4) )* ( 1 - (u-T/4) *4/T )"
  Fcn2 : Fcn  Expr=( (u > 3*T/4)&& (u<=T)) * ( ((u -3*T/4)* 4/T )-1 )
  Sum1 : Sum  Inputs=+++  OutDataType=sfix(16)  OutScaling=2^0
  O1 : Outport
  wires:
  I1/1 -> Fcn1/1, Fcn2/1, Fcn/1
  Sum1/1 -> O1/1
  Fcn/1 -> Sum1/1
  Fcn1/1 -> Sum1/2
  Fcn2/1 -> Sum1/3

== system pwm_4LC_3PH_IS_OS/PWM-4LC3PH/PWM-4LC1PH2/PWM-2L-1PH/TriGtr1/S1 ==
  I1 : Inport  OutDataType=sfix(16)  OutScaling=2^0
  Fcn : Fcn  Expr=u* (u <=T/4) * 4/T
  Fcn1 : Fcn  Expr="(  (u > T/4) && ( u <=3*T/4) )* ( 1 - (u-T/4) *4/T )"
  Fcn2 : Fcn  Expr=( (u > 3*T/4)&& (u<=T)) * ( ((u -3*T/4)* 4/T )-1 )
  Sum1 : Sum  Inputs=+++  OutDataType=sfix(16)  OutScaling=2^0
  O1 : Outport
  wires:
  Fcn2/1 -> Sum1/3
  Fcn1/1 -> Sum1/2
  Fcn/1 -> Sum1/1
  Sum1/1 -> O1/1
  I1/1 -> Fcn/1, Fcn2/1, Fcn1/1

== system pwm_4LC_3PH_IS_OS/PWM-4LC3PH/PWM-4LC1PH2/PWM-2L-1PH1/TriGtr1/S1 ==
  I1 : Inport  OutDataType=sfix(16)  OutScaling=2^0
  Fcn : Fcn  Expr=u* (u <=T/4) * 4/T
  Fcn1 : Fcn  Expr="(  (u > T/4) && ( u <=3*T/4) )* ( 1 - (u-T/4) *4/T )"
  Fcn2 : Fcn  Expr=( (u > 3*T/4)&& (u<=T)) * ( ((u -3*T/4)* 4/T )-1 )
  Sum1 : Sum  Inputs=+++  OutDataType=sfix(16)  OutScaling=2^0
  O1 : Outport
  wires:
  I1/1 -> Fcn1/1, Fcn2/1, Fcn/1
  Sum1/1 -> O1/1
  Fcn/1 -> Sum1/1
  Fcn1/1 -> Sum1/2
  Fcn2/1 -> Sum1/3

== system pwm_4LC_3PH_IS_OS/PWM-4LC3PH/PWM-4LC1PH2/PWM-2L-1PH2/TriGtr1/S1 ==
  I1 : Inport  OutDataType=sfix(16)  OutScaling=2^0
  Fcn : Fcn  Expr=u* (u <=T/4) * 4/T
  Fcn1 : Fcn  Expr="(  (u > T/4) && ( u <=3*T/4) )* ( 1 - (u-T/4) *4/T )"
  Fcn2 : Fcn  Expr=( (u > 3*T/4)&& (u<=T)) * ( ((u -3*T/4)* 4/T )-1 )
  Sum1 : Sum  Inputs=+++  OutDataType=sfix(16)  OutScaling=2^0
  O1 : Outport
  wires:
  Fcn2/1 -> Sum1/3
  Fcn1/1 -> Sum1/2
  Fcn/1 -> Sum1/1
  Sum1/1 -> O1/1
  I1/1 -> Fcn/1, Fcn2/1, Fcn1/1
